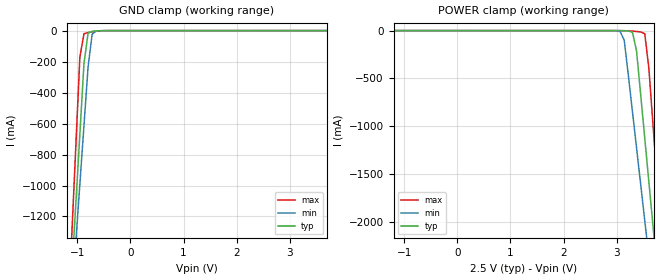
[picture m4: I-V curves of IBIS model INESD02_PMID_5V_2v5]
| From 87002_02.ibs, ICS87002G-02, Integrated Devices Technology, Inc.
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[Model] INESD02_PMID_5V_2v5
Model_type   Input
Polarity   Non-Inverting
Vinl = .8V
Vinh = 2V
|   typ   min   max
C_comp   2pF   1.5pF   2.5pF
|   typ   min   max
[Voltage range]  2.5V   2.375V   2.625V
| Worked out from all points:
|   GND clamp passes 1 mA (typ) near -0.59 V on its own axis
[GND_clamp]
|Voltage   I(typ)   I(min)   I(max)
-2.5V     -9.8A      -8.591A    -11.84A
-1.108V   -1.581A    -1.751A    -1.339A
-1.031V   -1.125A    -1.372A    -755.3mA
-953.6mV  -669.5mA   -992.5mA   -172.2mA
-876.3mV  -213.9mA   -613.8mA   -20.02mA
-799mV    -17.38mA   -235.4mA   -12.17mA
-721.6mV  -4.524mA   -23.09mA   -7.78mA
-644.3mV  -1.93mA    -2.602mA   -4.114mA
5V        157.2uA    199.8uA    119.8uA
[POWER_clamp]
|Voltage   I(typ)   I(min)   I(max)
-2.5V     157.2uA    193.3uA    123.8uA
2.835V    -69.15uA   -119.9uA   -49.49uA
3.067V    -682.6uA   -9.571mA   -166.6uA
3.144V    -1.93mA    -101.9mA   -694.4uA
3.299V    -17.38mA   -847.3mA   -5.416mA
3.376V    -213.9mA   -1.226A    -9.382mA
3.531V    -1.125A    -1.985A    -32.71mA
3.608V    -1.581A    -2.364A    -395.7mA
3.686V    -2.038A    -2.744A    -978.8mA
3.763V    -2.494A    -3.124A    -1.562A
3.84V     -2.95A     -3.504A    -2.145A
5V        -9.8A      -9.206A    -10.89A
